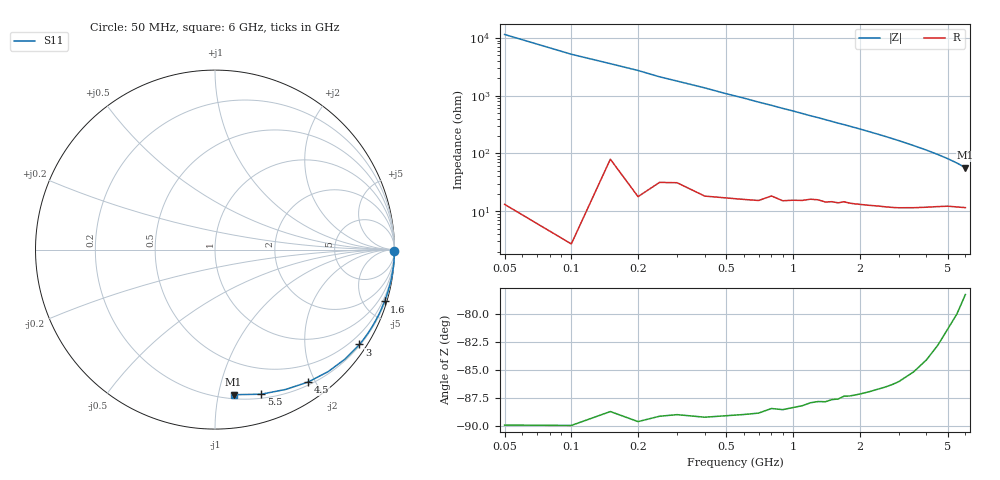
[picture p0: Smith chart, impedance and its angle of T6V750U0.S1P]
! SIEMENS Discrete & RF Semiconductors
! BAT62
! Si Schottky Diode in SOT143
! VR = 0.75 V
! S-Parameters:  February  1997
# GHz  S  MA  R  50
!  f  S11
! GHz  MAG  ANG
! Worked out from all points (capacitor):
!   34 points, 50 MHz to 6 GHz, reference 50 ohm
!   read as one part to ground: C = 296 fF near 50 MHz
!   lowest |Z| = 56.7 ohm at 6 GHz (marker M1)
!   S11 on the Smith chart (normalised r, x): 50 MHz: open; 1.6 GHz: 0.28, -6.68; 3 GHz: 0.23, -3.33; 4.5 GHz: 0.24, -1.91; 5.5 GHz: 0.24, -1.34; 6 GHz: 0.23, -1.11
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0.05  1 -0.5
0.1  1 -1.1
0.2  0.9998 -2.1
0.25  0.9993 -2.7
0.4  0.999 -4.2
0.5  0.9986 -5.3
0.6  0.9981 -6.3
0.7  0.9974 -7.4
0.8  0.9961 -8.4
0.9  0.9959 -9.5
1  0.9948 -10.5
1.1  0.9937 -11.6
1.4  0.9905 -14.8
1.6  0.9879 -17.0
1.7  0.9858 -18.0
1.8  0.9849 -19.1
2  0.9822 -21.3
2.2  0.979 -23.6
2.4  0.9755 -25.9
2.6  0.9718 -28.3
2.8  0.9676 -30.8
3  0.9629 -33.3
3.5  0.9474 -40.0
4  0.9274 -47.1
4.5  0.9022 -54.8
5  0.8733 -63.1
5.5  0.8458 -72.3
6  0.815 -82.7
